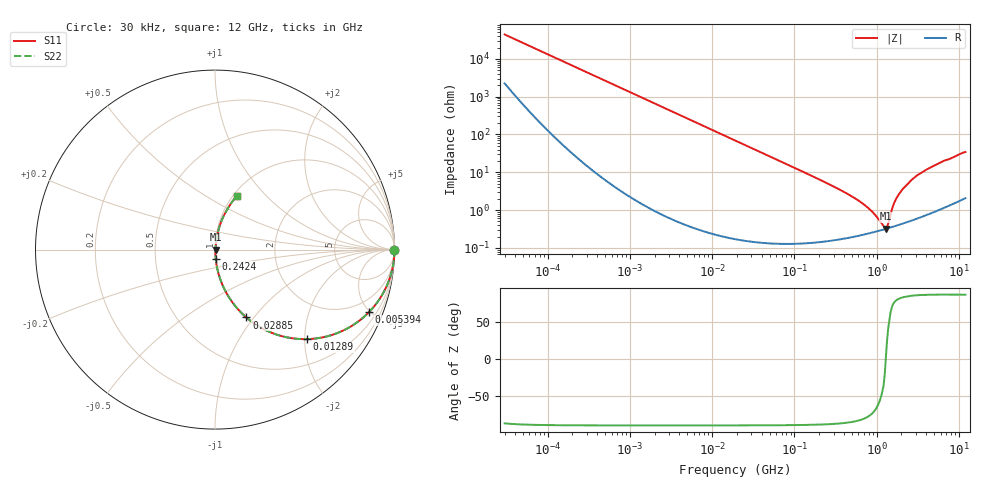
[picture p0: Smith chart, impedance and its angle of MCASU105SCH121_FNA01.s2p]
! MCASU105SCH121_FNA01  S-PARAMETER MODEL  ( General Type )
! Model Generated by TAIYO YUDEN Corporation (http://www.ty-top.com)
! Version 1.0
! TAIYO YUDEN Control No. 130207
! Copyright(c) 2013 TAIYO YUDEN CO.,LTD. All Rights Reserved.
! Product Description (link to TY-COMPAS)
! https://ds.yuden.co.jp/TYCOMPAS/or/detail?pn=MCASU105SCH121JFNA01&u=M
! Products Name : Multilayer Ceramic Capacitors
! Characteristics :
!  Capacitance : 120 pF , Rated Voltage : 50V , TCC : CH / C0H
!  Case Size : 1.0 x 0.5 / 0.039 x 0.02 [mm/inch] , Thickness : 0.5 / 0.02 [mm/inch]
!  (Conditions: Temperature = 25 degC , DC Bias Current/Voltage = 0A / 0V)
! External Node Assignments :
!  1  o---| |---o  2
! GND o---------o GND
! Frequency Range : 30000Hz  -  12GHz  [ 401 STEP ]
# MHz S RI R 50
! Freq[MHz].  S11 Real  S11 Imag  S21 Real  S21 Imag  S12 Real  S12 Imag  S22 Real  S22 Imag
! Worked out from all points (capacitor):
!   401 points, 30 kHz to 12 GHz, reference 50 ohm
!   read as one part in series: C = 120 pF near 32 kHz
!   lowest |Z| = 319 mohm at 1.297 GHz (marker M1)
!   series resonance near 1.292 GHz, so ESL is about 130 pH
!   S11 on the Smith chart (normalised r, x): 30 kHz: open; 5.394 MHz: 1.01, -4.91; 12.89 MHz: 1.00, -2.06; 28.85 MHz: 1.00, -0.92; 242.4 MHz: 1.00, -0.11; 12 GHz: 1.04, +0.69
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0.03  0.9999 -0.00226  0.00012 0.00226  0.00012 0.00226  0.9999 -0.00226
0.260295  0.9995 -0.0196  0.000459 0.0196  0.000459 0.0196  0.9995 -0.0196
0.915519  0.9951 -0.0687  0.00487 0.0687  0.00487 0.0687  0.9951 -0.0687
2.258455  0.9716 -0.1655  0.0284 0.1655  0.0284 0.1655  0.9716 -0.1655
5.39449  0.8575 -0.3488  0.1425 0.3488  0.1425 0.3488  0.8575 -0.3488
12.88515  0.5141 -0.4988  0.4859 0.4988  0.4859 0.4988  0.5141 -0.4988
18.97367  0.3283 -0.4684  0.6717 0.4684  0.6717 0.4684  0.3283 -0.4684
28.85481  0.1749 -0.3783  0.8251 0.3783  0.8251 0.3783  0.1749 -0.3783
56.79713  0.0526 -0.2204  0.9474 0.2204  0.9474 0.2204  0.0526 -0.2204
164.6252  0.00759 -0.0786  0.9924 0.0786  0.9924 0.0786  0.00759 -0.0786
242.4142  0.00426 -0.0526  0.9957 0.0526  0.9957 0.0526  0.00426 -0.0526
658.7456  0.00241 -0.0153  0.9976 0.0153  0.9976 0.0153  0.00241 -0.0153
909.4299  0.00264 -0.00803  0.9974 0.00803  0.9974 0.00803  0.00264 -0.00803
1215.67  0.00306 -0.00221  0.9969 0.00221  0.9969 0.00221  0.00306 -0.00221
1296.659  0.00318 0.00015  0.9968 -0.00015  0.9968 -0.00015  0.00318 0.00015
1428.372  0.0034 0.00427  0.9966 -0.00427  0.9966 -0.00427  0.0034 0.00427
1625.032  0.00389 0.0145  0.9961 -0.0145  0.9961 -0.0145  0.00389 0.0145
1790.1  0.00443 0.0223  0.9956 -0.0223  0.9956 -0.0223  0.00443 0.0223
2103.309  0.00574 0.0365  0.9943 -0.0365  0.9943 -0.0365  0.00574 0.0365
2722.352  0.00955 0.0646  0.9905 -0.0646  0.9905 -0.0646  0.00955 0.0646
5715.613  0.0383 0.1653  0.9617 -0.1653  0.9617 -0.1653  0.0383 0.1653
12000  0.1198 0.2961  0.8802 -0.2961  0.8802 -0.2961  0.1198 0.2961
